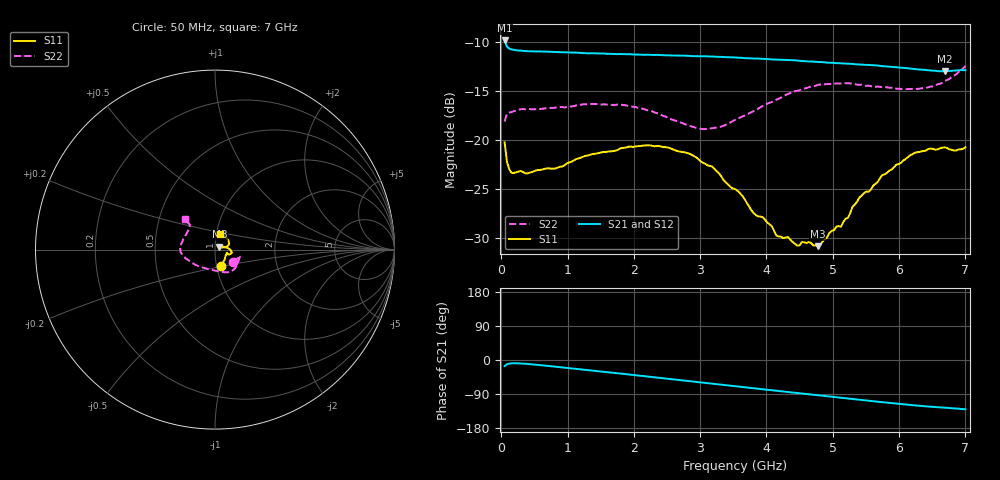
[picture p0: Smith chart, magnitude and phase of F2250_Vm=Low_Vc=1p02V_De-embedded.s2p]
! Integrated Device Technology
! Corporate Headquarters
! 6024 Silver Creek Valley Road
! San Jose, CA 95138  USA
! Phone:  1-408-284-8200
! Toll Free:  1-800-223-1366
! Webpage:  http://www.idt.com/
! Timing and RF Division
! 515 Groton Road, Suite 102
! Westford, MA 01886-6024
! Device:  F2250
! Description: Voltage Variable RF Attenuator
! Frequency:  50.0 -  6000.00 MHz
! Package:  3x3 mm Thin QFN Plastic Package: 16 pin
! Ports:  2 RF, 3 DC
!  Pin  1  = GND
!  Pin  2  = NC
!  Pin  3  = RF1  = Port 1
!  Pin  4  = NC
!  Pin  5  = GND
!  Pin  6  = GND
!  Pin  7  = GND
!  Pin  8  = GND
!  Pin  9  = NC
!  Pin 10  = RF2  = Port 2
!  Pin 11  = NC
!  Pin 12  = GND
!  Pin 13  = GND
!  Pin 14  = VCNTRL
!  Pin 15  = VDD
!  Pin 16  = VMODE
! Vcntrl:  1.020 Volts
! Vmode:  +0.000 Volts
! Vdd:  +3.30  Volts
! Current:  1.186 mA
! Data:  The device was measured on a the F2250 evaluation board which has
!  individual transmission lines to the RF pins.  Data was collected
!  using a calibrated network analyzer.  The evaluation board was
!  de-embedded using a TRL calibration technique.
!  The reference plane is the edge of the package pin.
! Misc:  SN 10
!  Action Tracker AT0258
! Date Measured:  2014-11-26
! Date:  2015-10-15  MJV
! Note:
!  Integrated Device Technology supplies this data as a sample of measured
!  data at the package pin for this product.  Your particular data for this
!  product may vary.
!  Data was taken at 25 degrees C.
!  Integrated Device Technology reserves the right to change this data at anytime.
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# GHz S dB R 50
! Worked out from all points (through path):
!   201 points, 50 MHz to 7 GHz, reference 50 ohm
!   highest |S21| = -9.83 dB at 50 MHz (marker M1); lowest = -13.0 dB at 6.687 GHz (marker M2)
!   group delay of S21, straight-line fit = 51.7 ps
!   lowest |S11| = -30.8 dB at 4.776 GHz (marker M3), VSWR 1.06, Z = 52.4 + j1.63 ohm
!   |S11| at or under -10 dB: start of sweep to end of sweep
!   |S22| runs from -18.9 to -12.4 dB; largest |S21 - S12| = 0.00073
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0.05  -20.23 -71.1  -9.83 -15.9  -9.82 -15.9  -18.10 -35.2
0.08475  -22.20 -46.1  -10.46 -11.4  -10.47 -11.4  -17.30 -19.6
0.15425  -23.34 -28.7  -10.74 -8.8  -10.74 -8.8  -17.14 -13.7
0.8145  -22.91 -16.5  -11.01 -17.6  -11.00 -17.6  -16.69 -29.4
1.2315  -21.70 -19.1  -11.11 -25.3  -11.11 -25.3  -16.36 -41.1
1.857  -20.79 -15.1  -11.23 -37.0  -11.22 -37.0  -16.43 -54.8
2.37825  -20.62 -8.6  -11.31 -46.8  -11.32 -46.8  -17.31 -67.9
3.0385  -22.31 3.3  -11.43 -59.6  -11.44 -59.6  -18.88 -99.8
3.525  -25.01 13.6  -11.57 -69.1  -11.58 -69.1  -17.94 -130.3
3.803  -27.43 23.0  -11.67 -74.4  -11.67 -74.5  -17.05 -144.1
4.081  -28.82 32.9  -11.77 -79.8  -11.77 -79.8  -16.11 -156.3
4.1505  -29.78 33.6  -11.78 -81.2  -11.78 -81.2  -15.88 -158.7
4.32425  -29.91 33.6  -11.83 -84.5  -11.85 -84.5  -15.30 -163.9
4.46325  -30.78 36.4  -11.89 -87.2  -11.90 -87.2  -14.97 -167.8
4.7065  -30.77 35.4  -11.99 -91.9  -11.98 -91.9  -14.52 -173.5
4.776  -30.84 32.7  -12.03 -93.2  -12.02 -93.2  -14.37 -175.0
5.1235  -28.86 21.7  -12.16 -99.8  -12.16 -99.8  -14.22 177.3
5.4015  -25.87 15.4  -12.28 -104.9  -12.28 -105.0  -14.34 170.8
5.85325  -23.13 15.2  -12.50 -113.1  -12.51 -113.2  -14.66 159.4
6.2355  -21.30 23.5  -12.75 -119.7  -12.74 -119.8  -14.79 146.8
6.68725  -20.74 45.3  -12.98 -125.8  -12.97 -125.8  -13.98 135.1
7  -20.74 73.5  -12.86 -130.1  -12.84 -130.2  -12.44 135.2
